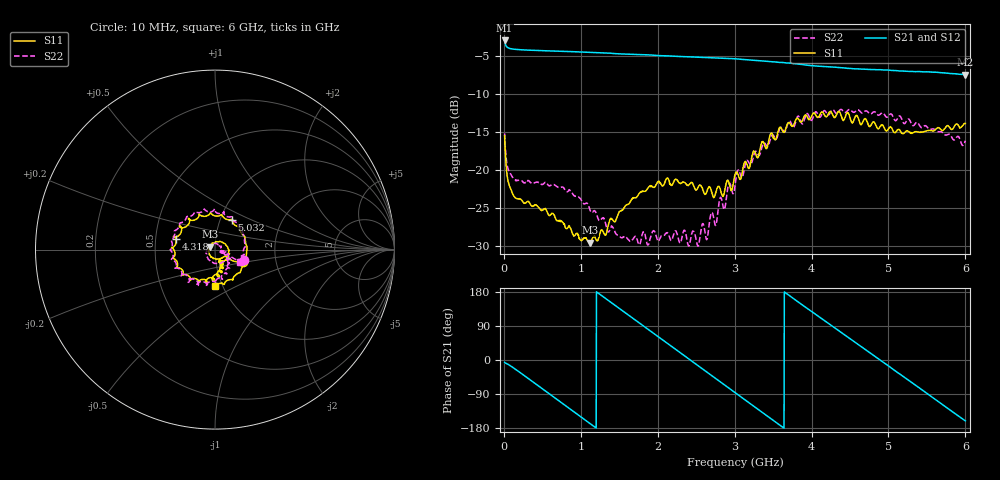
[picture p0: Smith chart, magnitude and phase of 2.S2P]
!Agilent Technologies,E5071C,MY46316741,A.11.02
!Date: Tue Oct 20 14:44:05 2020
!Data & Calibration Information:
!Freq	S11:SOLT4(ON)	S21:SOLT4(ON)	S12:SOLT4(ON)	S22:SOLT4(ON)
!PortZ  Port1:50+j0  Port2:50+j0
!Above PortZ is port z conversion or system Z0 setting when saving the data.
!When reading, reference impedance value at option line is always used.
# Hz S dB R 50
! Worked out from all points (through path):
!   1561 points, 10 MHz to 6 GHz, reference 50 ohm
!   highest |S21| = -2.95 dB at 10 MHz (marker M1); lowest = -7.5 dB at 6 GHz (marker M2)
!   group delay of S21, straight-line fit = 407 ps
!   lowest |S11| = -29.6 dB at 1.12 GHz (marker M3), VSWR 1.07, Z = 47.1 + j1.49 ohm
!   |S11| at or under -10 dB: start of sweep to end of sweep
!   |S22| runs from -30.0 to -12.0 dB; largest |S21 - S12| = 0.0048
!   S11 on the Smith chart (normalised r, x): 10 MHz: 1.35, -0.19; 4.318 GHz: 0.64, +0.08; 5.032 GHz: 1.13, +0.39; 6 GHz: 0.92, -0.39
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1e7  -15.51 -23.5  -2.95 -6.3  -3.00 -6.3  -15.19 -19.8
5.607692e7  -21.52 -32.3  -3.92 -11.6  -3.96 -11.6  -19.89 -23.7
1.290321e8  -23.41 -32.5  -4.10 -21.3  -4.14 -21.3  -21.15 -23.7
5.437244e8  -25.13 -82.5  -4.30 -82.2  -4.34 -82.2  -21.65 -64.6
7.664295e8  -26.89 -120.0  -4.38 -115.2  -4.41 -115.3  -22.25 -93.3
1.012173e9  -29.29 -177.3  -4.47 -151.7  -4.50 -151.8  -24.07 -129.5
1.119686e9  -29.57 151.6  -4.52 -167.6  -4.54 -167.7  -25.26 -148.2
1.346231e9  -27.77 88.0  -4.59 158.7  -4.62 158.6  -28.04 166.5
1.615013e9  -24.54 39.3  -4.76 119.2  -4.77 119.1  -29.13 101.8
2.006667e9  -21.49 -15.9  -4.94 61.4  -4.95 61.3  -29.38 18.1
2.248571e9  -21.28 -42.4  -5.04 25.8  -5.05 25.6  -28.32 -8.9
2.482795e9  -22.49 -58.4  -5.13 -8.5  -5.16 -8.8  -28.42 -13.2
2.640224e9  -22.80 -70.6  -5.19 -31.8  -5.22 -32.0  -29.14 -17.7
3.005e9  -20.62 -68.2  -5.36 -85.9  -5.41 -86.2  -22.10 -35.5
3.527205e9  -16.05 -97.0  -5.78 -163.0  -5.81 -163.1  -15.85 -78.6
4.007173e9  -12.75 -154.3  -6.26 127.2  -6.28 127.0  -13.38 -139.1
4.318192e9  -12.88 164.7  -6.48 82.3  -6.49 82.2  -12.54 -171.0
4.690647e9  -13.26 114.0  -6.73 29.1  -6.76 28.9  -12.28 144.0
5.001667e9  -14.56 63.1  -6.85 -16.1  -6.88 -16.1  -12.88 106.7
5.032385e9  -14.39 60.6  -6.89 -20.5  -6.91 -20.7  -12.61 104.8
5.512353e9  -14.81 -21.8  -7.08 -89.9  -7.09 -89.9  -14.47 46.9
6e9  -13.88 -90.3  -7.46 -160.8  -7.46 -160.7  -16.15 -27.1
